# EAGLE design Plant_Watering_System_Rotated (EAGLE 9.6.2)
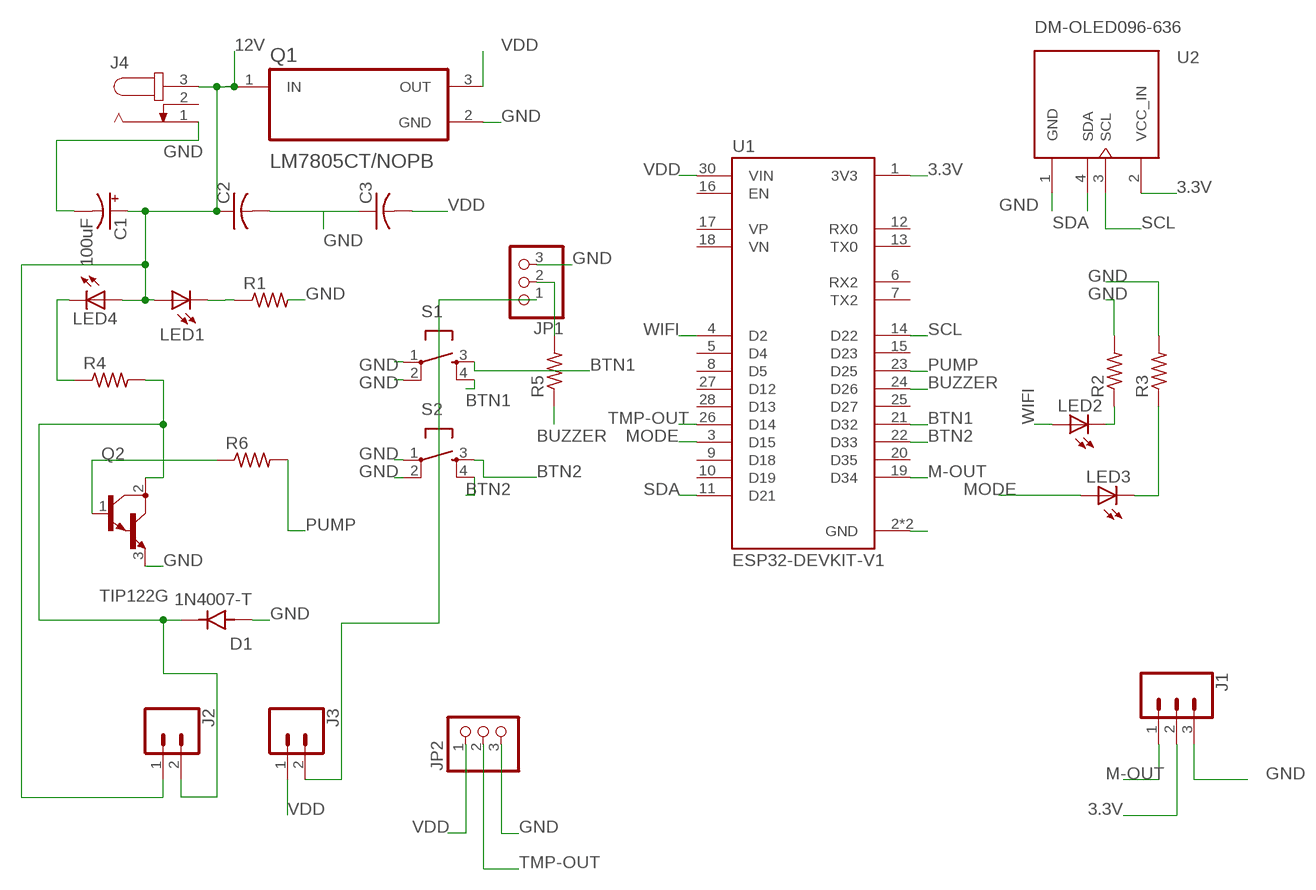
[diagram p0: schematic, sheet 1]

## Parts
C1  100uF  100UF-POLAR-RADIAL-2.5MM-25V-20%  [CPOL-RADIAL-2.5MM-6.5MM]
C2  C-US050-025X075  [C050-025X075]
C3  C-US050-025X075  [C050-025X075]
D1  1N4007-T  [DIOAD780W78L463D236]
J1  CONN_03-SCREW-5MM  [SCREWTERMINAL-5MM-3]
J2  CONN_025MM  [SCREWTERMINAL-5MM-2]
J3  CONN_025MM  [SCREWTERMINAL-5MM-2]
J4  JACK-PLUG1  [SPC4078]
JP1  PINHD-1X3  [1X03]
JP2  PINHD-1X3  [1X03]
LED1  LED5MM  [LED5MM]
LED2  LED5MM  [LED5MM]
LED3  LED5MM  [LED5MM]
LED4  LED5MM  [LED5MM]
Q1  LM7805CT/NOPB  [TO254P1054X470X1955-3]
Q2  TIP122G  [TO254P1009X445X1985-3]
R1  R-US_0309/10  [0309/10]
R2  R-US_0309/10  [0309/10]
R3  R-US_0309/10  [0309/10]
R4  R-US_0309/10  [0309/10]
R5  R-US_0309/10  [0309/10]
R6  R-US_0309/10  [0309/10]
S1  TAC_SWITCHPTH  [TACTILE-PTH]
S2  TAC_SWITCHPTH  [TACTILE-PTH]
U1  ESP32-DEVKIT-V1  [MODULE_ESP32_DEVKIT_V1]
U2  DM-OLED096-636  [MODULE_DM-OLED096-636]

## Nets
3.3V: J1.2 U1.1(3V3) U2.2(VCC_IN)
12V: C1.1(+) C2.1 J2.1 J4.3 LED1.A LED4.A Q1.1(IN)
BTN1: S1.3 S1.4 U1.21(D32)
BTN2: S2.3 S2.4 U1.22(D33)
BUZZER: R5.1 U1.24(D26)
GND: C1.2(-) C2.2 C3.1 D1.A J1.3 J4.1 JP1.3 JP2.3 Q1.2(GND) Q2.3(E) R1.2 R2.2 R3.2 S1.1 S1.2 S2.1 S2.2 U1.2(GND) U1.29(GND) U2.1(GND)
M-OUT: J1.1 U1.19(D34)
MODE: LED3.A U1.3(D15)
N$2: JP1.2 R5.2
N$3: LED1.K(C) R1.1
N$4: LED2.K(C) R2.1
N$5: LED4.K(C) R4.1
N$6: D1.K J2.2 Q2.2(C) R4.2
N$7: Q2.1(B) R6.1
N$11: J3.2 JP1.1
N$14: LED3.K(C) R3.1
PUMP: R6.2 U1.23(D25)
SCL: U1.14(D22) U2.3(SCL)
SDA: U1.11(D21) U2.4(SDA)
TMP-OUT: JP2.2 U1.26(D14)
VDD: C3.2 J3.1 JP2.1 Q1.3(OUT) U1.30(VIN)
WIFI: LED2.A U1.4(D2)
Unconnected: J4.2 U1.5(D4) U1.6(RX2) U1.7(TX2) U1.8(D5) U1.9(D18) U1.10(D19) U1.12(RX0) U1.13(TX0) U1.15(D23) U1.16(EN) U1.17(VP) U1.18(VN) U1.20(D35) U1.25(D27) U1.27(D12) U1.28(D13)

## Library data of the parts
C1 = SparkFun-Capacitors:100UF-POLAR: 100µF polarized capacitors; PROD_ID: CAP-08439
C2 C3 = rcl:C-US: CAPACITOR, American symbol; SPICEPREFIX: C
D1 = 1N4007-T:1N4007-T: Check availability Check availability Check availability; AVAILABILITY: In Stock; CHECK_PRICES: https://www.snapeda.com/parts/1N4007/NTE+Electronics/view-part/?ref=eda; DESCRIPTION: Rectifier Silicon, 1000V, 1 A, DO-41 Case, Solder Leads, 1N Series | NTE Electronics Inc. 1N4007; MF: NTE Electronics, Inc.; MP: 1N4007; PACKAGE: DO-41 NTE Electronics; PRICE: None; SNAPEDA_LINK: https://www.snapeda.com/parts/1N4007/NTE+Electronics/view-part/?ref=snap
J1 = SparkFun-Connectors:CONN_03: Multi connection point. Often used as Generic Header-pin footprint for 0.1 inch spaced/style header connections On any of the 0.1 inch spaced packages, you can populate with these: Break Away Headers - Straight (PRT-00116) Break Away Male Headers - Right Angle (PRT-00553) Female Headers (PRT-00115)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; PROD_ID: CONN-10134; SF_SKU: PRT-08433
J2 J3 = SparkFun-Connectors:CONN_02: Multi connection point. Often used as Generic Header-pin footprint for 0.1 inch spaced/style header connections; SF_SKU: PRT-08432
J4 = con-jack:JACK-PLUG: DC POWER JACK Power Jack, DC, Right Angle, Through Hole, Rated 5A at 16VDC, PC Terminals Distributor: Farnell (www.Farnell.de) Drawing: 84N1161.pdf / 84N1162.pdf Manufacturer: SPC Technology (www.spctechnology.com) Type: SPC4077 / SPC 4078; OC_FARNELL: unknown; OC_NEWARK: unknown
JP1 JP2 = adafruit:PINHD-1X3: PIN HEADER
LED1-LED4 = adafruit:LED: LED
Q1 = LM7805CT_NOPB:LM7805CT/NOPB: Check availability; AVAILABILITY: In Stock; CHECK_PRICES: https://www.snapeda.com/parts/LM7805CT/Texas+Instruments/view-part/?ref=eda; DESCRIPTION: 1.5-A, 35-V, linear voltage regulator 3-TO-220 0 to 125; MF: Texas Instruments; MP: LM7805CT; PACKAGE: TO-220-3 Texas Instruments; PRICE: None; SNAPEDA_LINK: https://www.snapeda.com/parts/LM7805CT/Texas+Instruments/view-part/?ref=snap
Q2 = TIP122G:TIP122G: Bipolar (BJT) Transistor NPN - Darlington 100V 5A 2W Through Hole TO-220AB Check availability; AVAILABILITY: Not in stock; CHECK_PRICES: https://www.snapeda.com/parts/TIP122G/Rochester+Electronics/view-part/?ref=eda; DESCRIPTION: Bipolar (BJT) Transistor NPN - Darlington 100V 5A 2W Through Hole TO-220AB; MF: Rochester Electronics, LLC; MP: TIP122G; PACKAGE: Package; PRICE: None; SNAPEDA_LINK: https://www.snapeda.com/parts/TIP122G/Rochester+Electronics/view-part/?ref=snap
R1-R6 = rcl:R-US_: RESISTOR, American symbol; SPICEPREFIX: R
S1 S2 = SparkFun-Retired:TAC_SWITCH: Momentary Switch Button commonly used for reset or general input. Spark Fun Electronics SKU : COM-00097 SMT- SWCH-08247
U1 = ESP32-DEVKIT-V1:ESP32-DEVKIT-V1: Dual core, Wi-Fi: 2.4 GHz up to 150 Mbits/s,BLE (Bluetooth Low Energy) and legacy Bluetooth, 32 bits, Up to 240 MHz Check availability; AVAILABILITY: Not in stock; CHECK_PRICES: https://www.snapeda.com/parts/ESP32-DEVKIT-V1/Do+it/view-part/?ref=eda; DESCRIPTION: Dual core, Wi-Fi: 2.4 GHz up to 150 Mbits/s,BLE (Bluetooth Low Energy) and legacy Bluetooth, 32 bits, Up to 240 MHz; MF: Do it; MP: ESP32-DEVKIT-V1; PACKAGE: None; PRICE: None; SNAPEDA_LINK: https://www.snapeda.com/parts/ESP32-DEVKIT-V1/Do+it/view-part/?ref=snap
U2 = DM-OLED096-636:DM-OLED096-636: Check availability; AVAILABILITY: Not in stock; CHECK_PRICES: https://www.snapeda.com/parts/DM-OLED096-636/Display+Module/view-part/?ref=eda; DESCRIPTION: 0.96” 128 X 64 MONOCHROME GRAPHIC OLED DISPLAY MODULE - I2C; MF: Display Module; MP: DM-OLED096-636; PACKAGE: Package; PRICE: None; SNAPEDA_LINK: https://www.snapeda.com/parts/DM-OLED096-636/Display+Module/view-part/?ref=snap

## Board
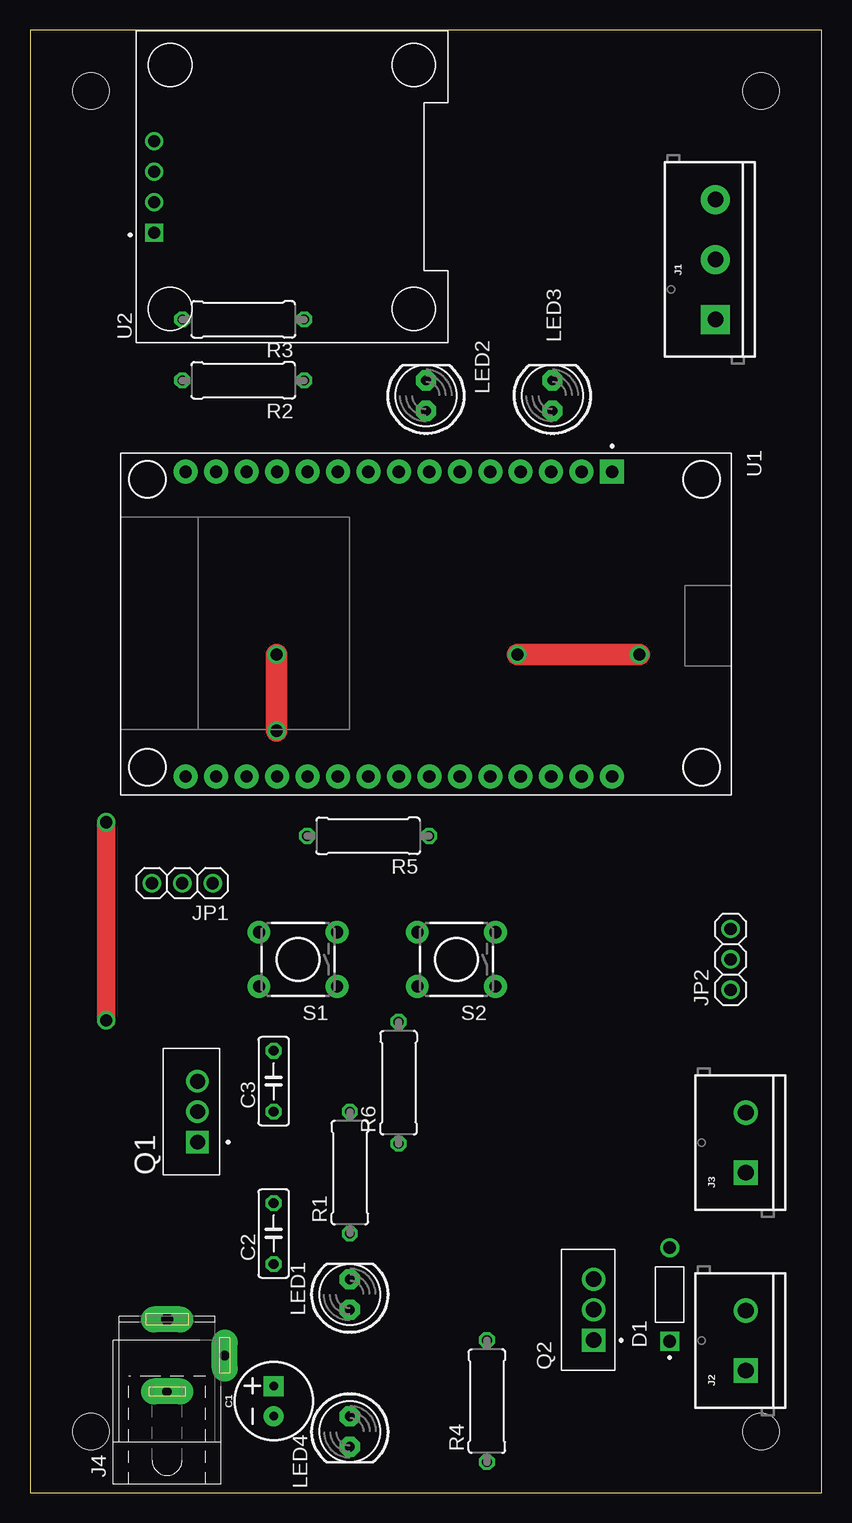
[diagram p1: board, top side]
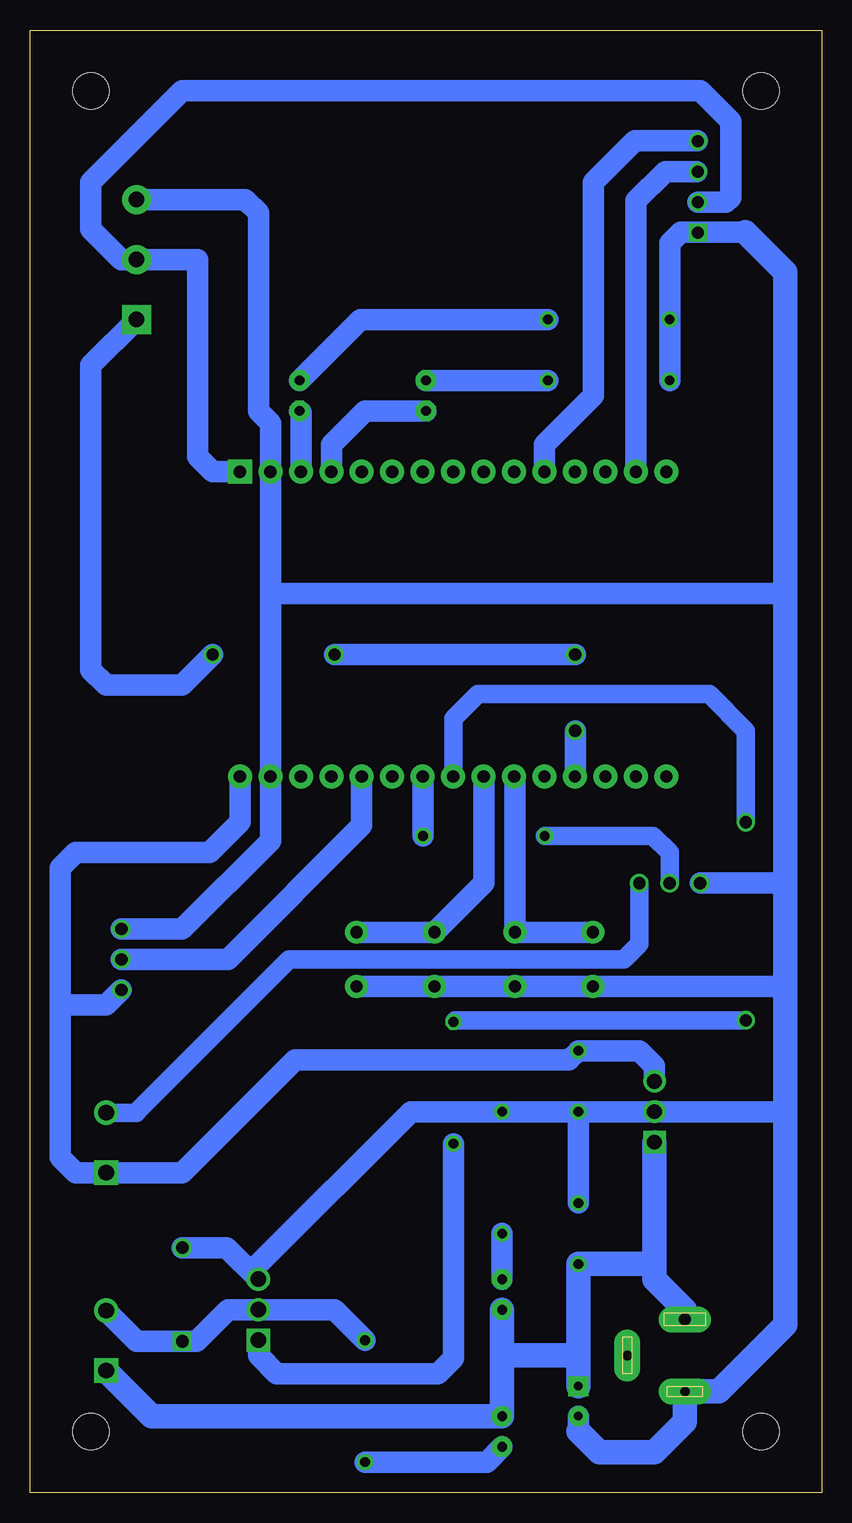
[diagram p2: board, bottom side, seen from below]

Size 66.04 x 121.92 mm. Coordinates in mm from the lower left corner, seen from the top.
Outline: 66.04,0 66.04,121.92 0,121.92 0,0 66.04,0
Copper layers (1*16): Top 0.035mm / dielectric 1.5mm / Bottom 0.035mm
Design rules "default": minimum track width 6mil, minimum drill 0.35mm, track to track 6mil, track to pad 6mil, pad to pad 6mil, via to via 6mil, smd to smd 6mil, copper to edge 40mil, drill to drill 6mil, minimum pad ring 10mil, minimum via ring 8mil, stop-mask expansion 4mil, vias tented up to drill 0mil, thermal gap 10mil
Holes 3.05 mm at 5.08,5.08 5.08,116.84 60.96,116.84 60.96,5.08

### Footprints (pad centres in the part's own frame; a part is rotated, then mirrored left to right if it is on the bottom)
CPOL-RADIAL-2.5MM-6.5MM = drill 0.7 pad 1.651 square: 1 1.25,0 | drill 0.7 pad 1.651: 2 -1.25,0
C050-025X075 = drill 0.813 octagon: 1 -2.54,0; 2 2.54,0
DIOAD780W78L463D236 = drill 1.06: A 3.905,0 | drill 1.06 square: K -3.905,0
SCREWTERMINAL-5MM-3 = drill 1.3 pad 2.413 square: 1 0,0 | drill 1.3 pad 2.413: 2 5,0; 3 10,0
SCREWTERMINAL-5MM-2 = drill 1.3 pad 2.032 square: 1 0,0 | drill 1.3 pad 2.032: 2 5,0
SPC4078 = drill 0.8 pad 2.184 long: 1 -3,0; 2 0,-4.8 | drill 1 pad 2.184 long: 3 3,0
1X03 = drill 1.016: 1 -2.54,0; 2 0,0; 3 2.54,0
LED5MM = drill 0.813 pad 1.676 octagon: A -1.27,0; K 1.27,0
TO254P1054X470X1955-3 = drill 1.24 square: 1 -2.54,0 | drill 1.24: 2 0,0; 3 2.54,0
TO254P1009X445X1985-3 = drill 1.29 pad 1.94 square: 1 -2.54,0 | drill 1.29 pad 1.94: 2 0,0; 3 2.54,0
0309/10 = drill 0.813 octagon: 1 -5.08,0; 2 5.08,0
TACTILE-PTH = drill 1.016 pad 1.88: 1 -3.251,2.261; 2 3.251,2.261; 3 -3.251,-2.261; 4 3.251,-2.261
MODULE_ESP32_DEVKIT_V1 = drill 1.02 pad 2 square: 1 -12.7,15.515 | drill 1.02 pad 2: 2 -12.7,12.975; 3 -12.7,10.435; 4 -12.7,7.895; 5 -12.7,5.355; 6 -12.7,2.815; 7 -12.7,0.275; 8 -12.7,-2.265; 9 -12.7,-4.805; 10 -12.7,-7.345; 11 -12.7,-9.885; 12 -12.7,-12.425; 13 -12.7,-14.965; 14 -12.7,-17.505; 15 -12.7,-20.045; 16 12.7,-20.045; 17 12.7,-17.505; 18 12.7,-14.965; 19 12.7,-12.425; 20 12.7,-9.885; 21 12.7,-7.345; 22 12.7,-4.805; 23 12.7,-2.265; 24 12.7,0.275; 25 12.7,2.815; 26 12.7,5.355; 27 12.7,7.895; 28 12.7,10.435; 29 12.7,12.975; 30 12.7,15.515
MODULE_DM-OLED096-636 = drill 1 square: 1 -3.81,11.5 | drill 1: 2 -1.27,11.5; 3 1.27,11.5; 4 3.81,11.5

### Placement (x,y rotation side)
C1  20.32,7.62 90 top
C2  20.32,21.59 90 top
C3  20.32,34.29 90 top
D1  53.34,16.51 90 top
J1  57.15,97.79 90 top
J2  59.69,10.16 90 top
J3  59.69,26.67 90 top
J4  11.43,11.43 90 top
JP1  12.7,50.8 180 top
JP2  58.42,44.45 90 top
LED1  26.67,16.51 90 top
LED2  33.02,91.44 90 top
LED3  43.56,91.44 90 top
LED4  26.67,5.08 270 top
Q1  13.97,31.75 90 top
Q2  46.99,15.24 90 top
R1  26.67,26.67 90 top
R2  17.78,92.71 180 top
R3  17.78,97.79 180 top
R4  38.1,7.62 90 top
R5  28.19,54.74 180 top
R6  30.73,34.16 90 top
S1  22.35,44.45 180 top
S2  35.56,44.45 180 top
U1  33.02,72.39 270 top
U2  21.84,108.84 90 top

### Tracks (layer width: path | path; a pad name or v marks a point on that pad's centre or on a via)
3.3V
  Bottom 0.152: U2.2 8,107.57
  Bottom 1.778: 10.36,107.57 8,107.57 7.62,107.95 7.62,114.3 10.16,116.84 53.34,116.84 60.96,109.22 60.96,105.33 58.42,102.79 J1.2 52.07,102.79 52.07,86.36 50.8,85.09 U1.1
12V
  Bottom 1.778: 26.67,11.43 LED1.A
  Bottom 2.032: Q1.1 13.97,19.05 | 13.97,19.05 13.97,17.78 11.43,15.24 J4.3 | 13.97,19.05 C2.1 | 19.05,19.05 C2.1 | C1.1 20.32,11.43 | 20.32,11.43 | 26.67,11.43 20.32,11.43 | LED1.A LED4.A 55.88,6.35 J2.1 | C2.1 20.32,11.43
BTN1
  Bottom 0.152: U1.21 25.6,59.62
  Bottom 1.778: S1.3 25.68,46.78 | S1.4 S1.3 | 25.6,59.62 S1.3
BTN2
  Bottom 0.152: U1.22 28.19,59.67
  Bottom 1.778: 28.19,59.67 28.19,50.83 S2.4 S2.3
BUZZER
  Bottom 0.152: U1.24 33.27,59.67
  Bottom 1.778: 33.27,59.67 R5.1
GND
  Bottom 0.152: 3.05,74.17 3.81,74.93 3.05,74.93 | 3.33,42.19 3.05,41.91 | 46.99,19.05 Q2.3 | U1.2 45.97,85.11 | 6.37,105.05 6.38,105.06 | 11.78,105.06 11.81,105.03 U2.1
  Bottom 1.778: S2.1 S2.2 S1.1 S1.2 3.33,42.19 | JP2.3 53.34,46.99 45.99,54.34 U1.29 45.99,74.93 | 20.32,5.1 C1.2 | R2.2 R3.2 12.7,104.14 11.81,105.03 | JP1.3 3.05,50.8 | 3.05,31.75 Q1.2 C3.1 | C3.1 R1.2 34.29,31.75 46.99,19.05 | Q2.3 49.62,20.41 D1.A | J1.3 48.1,107.79 46.99,106.68 46.99,90.17 45.97,89.15 45.97,85.11 | 45.99,74.93 U1.2 | 45.99,74.93 3.81,74.93 | C2.2 C3.1 | 6.38,105.06 11.78,105.06
  Bottom 2.032: 6.37,105.05 3.05,101.73 3.05,74.93 3.05,50.8 3.05,41.91 3.05,31.75 3.05,13.97 8.59,8.43 J4.1 11.43,5.89 13.97,3.35 18.57,3.35 20.32,5.1
M-OUT  (via drill 1.02)
  Top 1.778: v50.8,69.85 v40.64,69.85 | v20.57,69.85 v20.57,63.5
  Bottom 0.152: 20.57,59.71 U1.19
  Bottom 1.778: J1.1 60.96,93.98 60.96,68.58 59.69,67.31 53.34,67.31 v50.8,69.85 | v20.57,69.85 v40.64,69.85 | v20.57,63.5 20.57,59.71
MODE
  Bottom 0.152: LED3.A 43.43,90.04 | U1.3 43.43,85.11
  Bottom 1.778: LED3.A 43.45,90.06 | 43.43,90.04 43.43,85.11
N$2
  Bottom 1.524: JP1.2 12.7,53.34 14.1,54.74 R5.2
N$3
  Bottom 1.778: LED1.K R1.1
N$4
  Bottom 1.778: R2.1 LED2.K
N$5
  Bottom 1.778: LED4.K 27.94,2.54 R4.1
N$6
  Bottom 0.152: 49.44,15.24 52.07,12.61 D1.K | Q2.2 49.53,15.24
  Bottom 1.778: 49.44,15.24 40.64,15.24 R4.2 | J2.2 57.14,12.61 D1.K 52.16,12.61 49.53,15.24
N$7
  Bottom 1.778: Q2.1 46.99,11.43 45.47,9.91 32,9.91 30.73,11.18 R6.1
N$11
  Bottom 1.524: J3.2 57.15,31.67 57.19,31.71 44.45,44.45 16.51,44.45 15.24,45.72 JP1.1
N$14
  Bottom 1.778: R3.1 38.48,97.79 LED3.K
PUMP  (via drill 1.02)
  Top 1.524: v6.35,39.37 v6.35,55.88
  Bottom 0.152: 30.61,39.37 R6.2 | U1.23 30.73,59.71
  Bottom 1.524: v6.35,55.88 6.35,63.5 9.4,66.55 28.7,66.55 30.73,64.52 30.73,59.71 | v6.35,39.37 30.61,39.37
SCL
  Bottom 0.152: U2.3 13.08,110.11
  Bottom 1.778: 10.42,110.11 13.08,110.11 15.52,107.67 U1.14
SDA
  Bottom 0.152: 15.56,112.65 15.59,112.68 | 10.38,112.68 U2.4
  Bottom 1.778: U1.11 23.14,87.36 19.05,91.44 19.05,109.22 15.59,112.68 10.38,112.68
TMP-OUT
  Bottom 1.778: JP2.2 49.53,44.45 38.38,55.6 U1.26
VDD
  Bottom 1.778: 63.5,40.64 63.5,27.94 62.23,26.67 J3.1 53.34,26.67 43.94,36.07 21.08,36.07 C3.2 15.24,36.83 13.97,35.56 Q1.3 | 63.5,40.64 63.5,52.07 62.23,53.34 51.08,53.34 48.53,55.88 U1.30 | JP2.1 59.69,40.64 63.5,40.64
WIFI
  Bottom 1.778: LED2.A 38.1,90.17 40.91,87.36 U1.4

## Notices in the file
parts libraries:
SparkFun-Capacitors: Licensing: Creative Commons ShareAlike 4.0 International - https://creativecommons.org/licenses/by-sa/4.0
